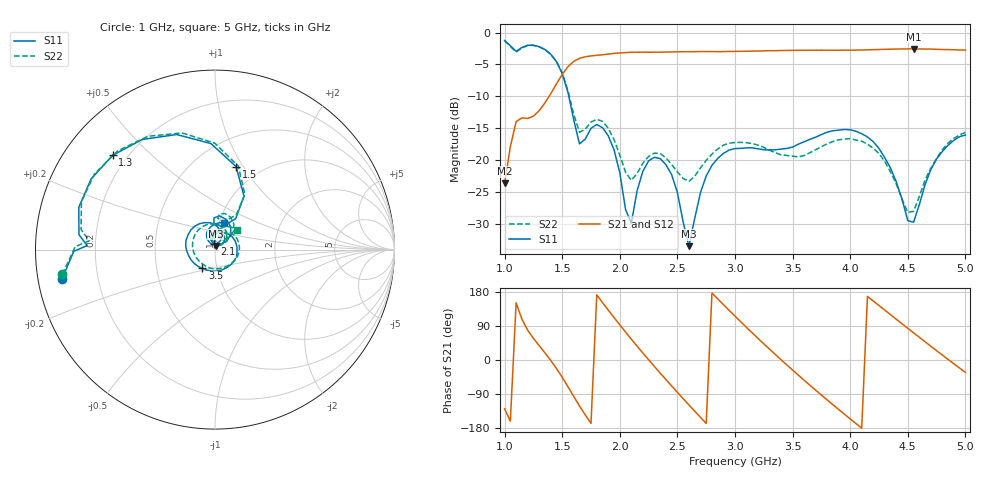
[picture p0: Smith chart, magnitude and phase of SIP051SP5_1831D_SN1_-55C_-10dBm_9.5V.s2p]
# GHz  S  dB  R  50
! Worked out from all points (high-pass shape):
!   81 points, 1 GHz to 5 GHz, reference 50 ohm
!   highest |S21| = -2.56 dB at 4.55 GHz (marker M1); lowest = -23.7 dB at 1 GHz (marker M2)
!   |S21| within 3 dB of the highest: 1.542 GHz to end of sweep
!   lowest |S11| = -33.5 dB at 2.6 GHz (marker M3), VSWR 1.04, Z = 50.5 + j2.06 ohm
!   |S11| at or under -10 dB: 1.557 GHz to end of sweep
!   |S22| runs from -28.2 to -1.3 dB; largest |S21 - S12| = 0.0026
!   S11 on the Smith chart (normalised r, x): 1 GHz: 0.07, -0.09; 1.3 GHz: 0.15, +0.38; 1.5 GHz: 0.78, +0.93; 2.1 GHz: 0.99, +0.06; 3.5 GHz: 0.85, -0.18; 5 GHz: 1.06, +0.32
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1  -1.25 -169.3  -23.67 -128.9  -23.72 -128.6  -1.29 -170.8
1.1  -2.94 178.2  -13.98 150.9  -14.00 150.9  -3.07 176.0
1.3  -2.21 137.4  -12.27 37.9  -12.26 38.0  -2.25 134.6
1.5  -6.43 75.7  -6.58 -45.6  -6.58 -45.6  -6.33 74.4
1.6  -13.70 56.2  -4.53 -96.1  -4.52 -96.2  -12.84 58.4
1.7  -16.73 92.4  -3.81 -144.8  -3.80 -144.9  -15.17 84.9
1.8  -14.44 82.5  -3.58 171.8  -3.58 171.8  -13.62 74.9
1.95  -18.42 43.2  -3.28 112.0  -3.28 112.1  -16.81 44.5
2.1  -29.91 96.8  -3.10 55.0  -3.10 55.0  -23.20 63.6
2.2  -21.79 106.8  -3.08 18.4  -3.09 18.5  -20.52 77.4
2.35  -19.78 70.0  -3.08 -34.3  -3.08 -34.2  -18.98 58.5
2.6  -33.54 76.0  -3.01 -118.6  -3.00 -118.7  -23.35 57.2
2.8  -20.85 84.2  -2.99 177.0  -2.98 177.0  -19.08 58.9
3  -18.22 22.4  -2.97 115.6  -2.96 115.7  -17.26 25.0
3.3  -18.43 -72.1  -2.85 28.6  -2.87 28.6  -18.49 -42.3
3.5  -17.99 -124.3  -2.80 -26.5  -2.80 -26.6  -19.42 -104.3
3.7  -16.43 -167.7  -2.78 -79.6  -2.78 -79.6  -18.41 -173.3
4.05  -15.49 120.4  -2.76 -167.7  -2.75 -167.7  -16.89 93.7
4.35  -21.27 64.0  -2.62 119.6  -2.63 119.7  -21.88 38.4
4.55  -29.78 109.0  -2.56 71.7  -2.58 71.8  -28.07 75.5
4.8  -18.68 109.5  -2.67 13.0  -2.67 13.1  -18.38 76.7
5  -16.10 70.5  -2.75 -32.6  -2.76 -32.6  -15.67 41.9
